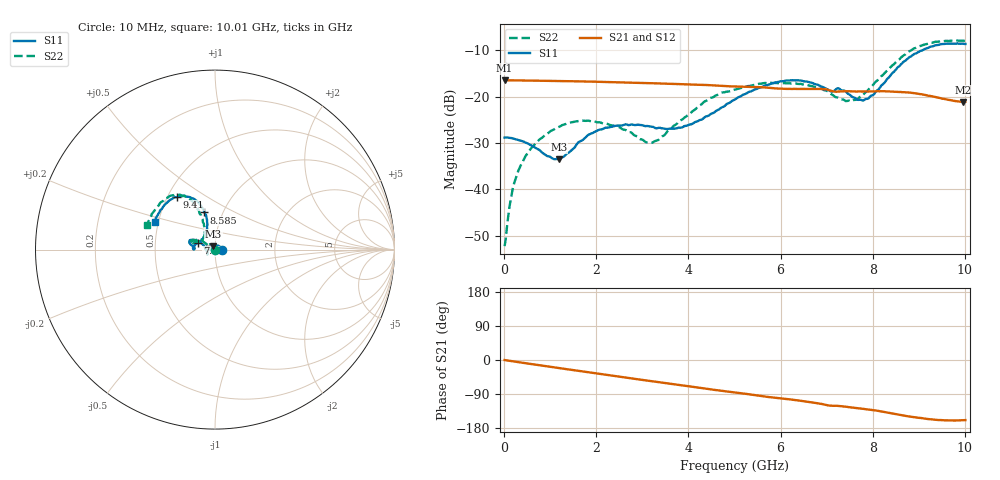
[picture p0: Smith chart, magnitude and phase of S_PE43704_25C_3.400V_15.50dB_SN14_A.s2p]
! Device ID: PE43704
! Dir: z:\PE43704\PE43704_Char_1_20130516\PE43704\AMB\3p400V\15p50dB
! Serial: 14
! Insertion: A
! Impedance: 50 ohm
! Temp: Amb
! VDD: 3.400V
! Attenuation Step: 15.50dB
! IDD: 1.139975e-01mA
#  Hz  S  RI  R  50
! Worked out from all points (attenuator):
!   401 points, 10 MHz to 10.01 GHz, reference 50 ohm
!   highest |S21| = -16.45 dB at 10 MHz (marker M1); lowest = -21.2 dB at 9.96 GHz (marker M2)
!   lowest |S11| = -33.5 dB at 1.185 GHz (marker M3), VSWR 1.04, Z = 49 + j1.84 ohm
!   |S11| at or under -10 dB: start of sweep to 9.075 GHz
!   |S22| runs from -52.3 to -7.9 dB; largest |S21 - S12| = 0.0011
!   S11 on the Smith chart (normalised r, x): 10 MHz: 1.08, +0.00; 7.51 GHz: 0.82, +0.06; 8.585 GHz: 0.82, +0.36; 9.41 GHz: 0.56, +0.38; 10.01 GHz: 0.48, +0.17
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1e7  0.0362 0.00028  0.1505 -0.000535  0.1506 -0.000496  -0.00239 0.000495
1.85e8  0.0347 0.00725  0.1498 -0.00901  0.1498 -0.00898  -0.00269 0.00975
3.6e8  0.0308 0.0132  0.1488 -0.0172  0.1488 -0.0175  -0.00593 0.0172
7.1e8  0.0168 0.0219  0.1452 -0.0331  0.1451 -0.033  -0.0174 0.0274
1.185e9  -0.00973 0.0188  0.1377 -0.0533  0.1378 -0.0532  -0.0391 0.0264
1.685e9  -0.0335 0.00262  0.1267 -0.0728  0.1268 -0.0727  -0.054 0.0121
2.41e9  -0.0438 -0.0207  0.1059 -0.0968  0.1059 -0.0967  -0.0477 -0.00335
3.11e9  -0.0413 -0.025  0.0818 -0.1141  0.0819 -0.1141  -0.0316 0.00579
3.36e9  -0.0414 -0.0204  0.0723 -0.1187  0.0724 -0.1186  -0.0317 0.0137
4.035e9  -0.0502 0.00295  0.0464 -0.127  0.0465 -0.1268  -0.0547 0.0366
4.46e9  -0.0604 0.0202  0.0301 -0.1298  0.0302 -0.13  -0.0787 0.0552
5.01e9  -0.0841 0.0408  0.00976 -0.1286  0.00991 -0.1287  -0.1071 0.0525
5.96e9  -0.134 0.0548  -0.0229 -0.1203  -0.0224 -0.1205  -0.1342 0.0404
6.685e9  -0.1377 0.0303  -0.0453 -0.1127  -0.0453 -0.1126  -0.1258 0.033
7.51e9  -0.0972 0.037  -0.0654 -0.0938  -0.0654 -0.0939  -0.0678 0.0584
7.86e9  -0.0626 0.0713  -0.0732 -0.0874  -0.0729 -0.0873  -0.057 0.0973
8.36e9  -0.0443 0.1578  -0.0868 -0.0737  -0.0862 -0.0739  -0.0766 0.186
8.585e9  -0.0596 0.2072  -0.0917 -0.0649  -0.091 -0.0652  -0.1012 0.234
8.935e9  -0.1051 0.2736  -0.0957 -0.0513  -0.0955 -0.0509  -0.163 0.2948
9.41e9  -0.2108 0.2928  -0.0907 -0.0363  -0.0907 -0.036  -0.2628 0.2904
9.96e9  -0.329 0.1777  -0.0817 -0.0314  -0.0824 -0.0313  -0.3716 0.156
1.001e10  -0.3365 0.1558  -0.0819 -0.0321  -0.0819 -0.0321  -0.3763 0.1363
